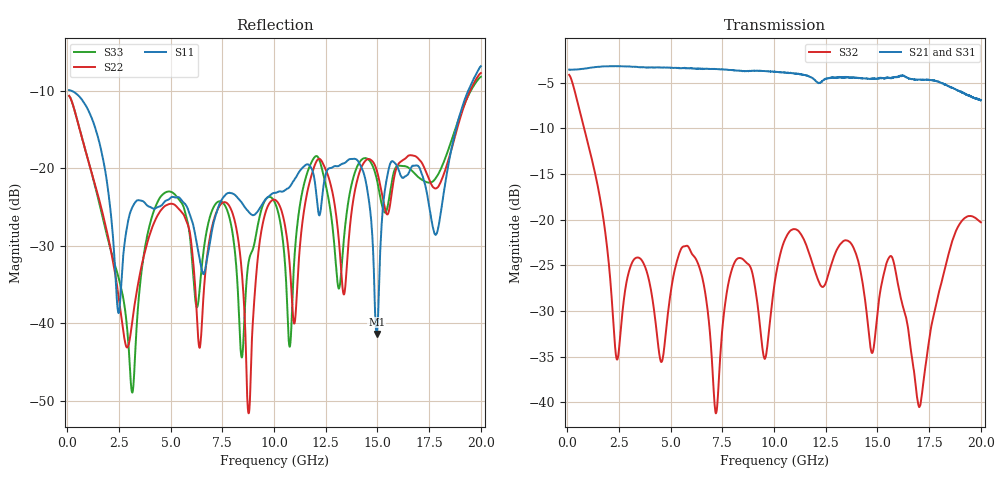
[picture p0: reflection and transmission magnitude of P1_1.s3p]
!The following data was pulled from an Agilent PNA
!This sNp file was generated from the data in the RF Test software
!NOTE:  Smoothing/Math/Corrections applied on any given trace ARE included in the data saved here
# MHz S dB R 50
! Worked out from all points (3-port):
!   6401 points, 100 MHz to 20 GHz, reference 50 ohm
!   strongest paths, dB at 100 MHz, 5.075 GHz, 10.05 GHz, 15.03 GHz, 20 GHz:
!     S21: -3.6, -3.4, -3.8, -4.5, -6.9
!     S31: -3.6, -3.4, -3.9, -4.5, -6.7
!     S32: -4.1, -27.0, -26.7, -29.7, -20.3
!   lowest |S11| = -41.4 dB at 14.97 GHz (marker M1), VSWR 1.02, Z = 50.8 + j0.145 ohm
!   |S11| at or under -10 dB: 236.3 MHz to 19.38 GHz (19.15 GHz wide, 195 % of centre)
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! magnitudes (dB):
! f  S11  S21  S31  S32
! 100 MHz  -9.9  -3.6  -3.6  -4.1
! 3.147 GHz  -25.1  -3.3  -3.3  -24.7
! 4.416 GHz  -25.0  -3.3  -3.3  -34.0
! 7.709 GHz  -23.3  -3.6  -3.6  -28.1
! 8.775 GHz  -25.6  -3.7  -3.8  -24.9
! 10.05 GHz  -23.1  -3.8  -3.9  -26.7
! 10.76 GHz  -22.4  -3.9  -4.0  -21.3
! 11.86 GHz  -20.3  -4.5  -4.6  -24.8
! 14.97 GHz  -41.4  -4.6  -4.5  -30.8
! 20 GHz  -6.8  -6.9  -6.7  -20.3
